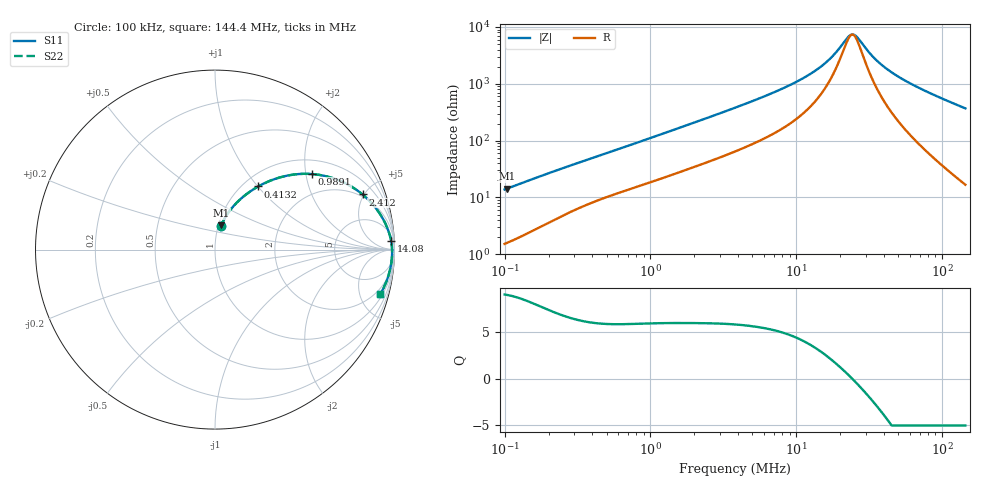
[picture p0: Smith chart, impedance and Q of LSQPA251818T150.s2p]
! LSQPA251818T150  S-PARAMETER MODEL  ( General Type )
! Model Generated by TAIYO YUDEN Corporation (http://www.ty-top.com)
! Version 2.0
! TAIYO YUDEN Control No. 100810NF25SB-FAC
! Copyright(c) 2007 TAIYO YUDEN CO.,LTD. All Rights Reserved.
! Product Description (link to TY-COMPAS)
! https://ds.yuden.co.jp/TYCOMPAS/or/detail?pn=LSQPA251818T150K&u=M
! Products Name : Inductors
! Characteristics :
!  Inductance : 15 uH , SRF(min) : 23 MHz , DC Resistance(max) : 0.845 Ohm
!  Rated Current : Saturation :350 mA , Temp Rise : 500 mA (40 degC)
!  Case Size : 2.5 x 1.8 / 0.098 x 0.071 [mm/inch] , Thickness : 1.8 / 0.071 [mm/inch]
!  (Conditions: Temperature = 25 degC , DC Bias Current/Voltage = 0A / 0V)
! External Node Assignments :
!  1  o---GGG---o  2
! GND o---------o GND
! Frequency Range : 0.1MHz  -  144.390904MHz  [ 402 STEP ]
# MHz S RI R 50
! Freq[MHz].  S11 Real  S11 Imag  S21 Real  S21 Imag  S12 Real  S12 Imag  S22 Real  S22 Imag
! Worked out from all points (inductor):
!   401 points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, 100 kHz to 144.4 MHz, reference 50 ohm
!   read as one part in series: L = 21.6 uH near 103.7 kHz
!   highest Q = 8.96 at 103.7 kHz (marker M1), where L = 21.8 uH
!   self-resonance near 24.19 MHz
!   S11 on the Smith chart (normalised r, x): 100 kHz: 1.03, +0.27; 413.2 kHz: 1.17, +1.01; 989.1 kHz: 1.37, +2.17; 2.412 MHz: 1.82, +4.87; 14.08 MHz: 12, +35; 144.4 MHz: 1.34, -7.38
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0.1  0.0327 0.1307  0.9673 -0.1307  0.9673 -0.1307  0.0327 0.1307
0.103705  0.0345 0.135  0.9655 -0.135  0.9655 -0.135  0.0345 0.135
0.192468  0.0885 0.2248  0.9115 -0.2248  0.9115 -0.2248  0.0885 0.2248
0.338238  0.1904 0.32  0.8096 -0.32  0.8096 -0.32  0.1904 0.32
0.413152  0.2409 0.3519  0.7591 -0.3519  0.7591 -0.3519  0.2409 0.3519
0.662949  0.3906 0.4097  0.6094 -0.4097  0.6094 -0.4097  0.3906 0.4097
0.989134  0.5409 0.4209  0.4591 -0.4209  0.4591 -0.4209  0.5409 0.4209
1.144052  0.5959 0.4137  0.4041 -0.4137  0.4041 -0.4137  0.5959 0.4137
2.411563  0.8221 0.3074  0.1779 -0.3074  0.1779 -0.3074  0.8221 0.3074
3.869624  0.9035 0.2213  0.0965 -0.2213  0.0965 -0.2213  0.9035 0.2213
7.865456  0.9624 0.1147  0.0376 -0.1147  0.0376 -0.1147  0.9624 0.1147
12.85266  0.9792 0.0592  0.0208 -0.0592  0.0208 -0.0592  0.9792 0.0592
14.07625  0.981 0.0501  0.019 -0.0501  0.019 -0.0501  0.981 0.0501
17.83085  0.9845 0.0276  0.0155 -0.0276  0.0155 -0.0276  0.9845 0.0276
22.58693  0.9863 0.00616  0.0137 -0.00616  0.0137 -0.00616  0.9863 0.00616
24.2914  0.9866 -0.000387  0.0134 0.000387  0.0134 0.000387  0.9866 -0.000387
26.1245  0.9868 -0.00696  0.0132 0.00696  0.0132 0.00696  0.9868 -0.00696
34.94858  0.9863 -0.0341  0.0137 0.0341  0.0137 0.0341  0.9863 -0.0341
43.47261  0.9846 -0.0562  0.0154 0.0562  0.0154 0.0562  0.9846 -0.0562
54.07568  0.9813 -0.0808  0.0187 0.0808  0.0187 0.0808  0.9813 -0.0808
71.03701  0.9741 -0.1165  0.0259 0.1165  0.0259 0.1165  0.9741 -0.1165
144.3909  0.922 -0.2465  0.078 0.2465  0.078 0.2465  0.922 -0.2465
